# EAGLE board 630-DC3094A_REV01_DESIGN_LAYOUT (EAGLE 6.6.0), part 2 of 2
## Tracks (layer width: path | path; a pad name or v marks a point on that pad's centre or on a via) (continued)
N$30  (via drill 0.2) (continued)
  Bottom 0.15: v204.8,77 204.8,76.3 205,76.1 205.68,76.1
PFET_GATE
  Bottom 0.1: 21.3,73.4 M3.1 21.2,73.45 21.2,74.2 21.4,74.4 22.6,74.4 | 25.3,73.48 M2.1 | M1.1 29.3,73.52 29.3,74.2 29.1,74.4 25.5,74.4 25.3,74.2 | 25.3,74.2 M2.1 | M2.1 25.29,74.11 25.3,74.2 | 25.3,74.2 25.1,74.4 22.6,74.4 | 22.6,74.4 22.6,69.9 22.56,69.94 R10.1
  Bottom 0.15: R9.2 R10.1
PWRGD  (via drill 0.2)
  Top 0.1: U1.R1 129.3,54.8 129.3,57 128.9,57.4 v128.9,60.2 | v140.1,55.2 U1.A1 | U1.H1 v134.5,55.2
  Route2 0.1: v128.9,60.2 v133.7,60.2 v140.1,60.2 v160.4,60.2
  Route15 0.1: v140.1,60.2 v140.1,55.2 | v134.5,55.2 134.5,56.2 134.1,56.6 134.1,59.8 v133.7,60.2 | v160.4,60.2 160.41,77.2 161,77.8 161,81.05 TP8.TP
  Bottom 0.1: M4.1 165.4,77.05 R54.1 165.41,77.2 165.41,80.2 164.41,81.2 161.61,81.2 TP8.TP
  pour Route15 (no thermals): 161,78.6 160.9,79.2 160.6,79.7 161.4,79.7 161.1,79.2
  pour Bottom (no thermals): 163.81,81.2 163.21,81.3 162.81,81.6 162.81,80.8 163.21,81.1
PWRGD_A
  Top 0.152: J1.49 17.14,11.43 17.14,17.78 J7.49
PWRGD_B
  Top 0.152: J2.49 105.41,11.43 105.41,17.78 J8.49
PWRGD_C
  Top 0.152: J3.49 193.68,11.43 193.68,17.78 J9.49
REFM_A  (via drill 0.2)
  Top 0.1: U1.G1 v135.3,55.2 | 139,68.2 C10.2
  Top 0.15: v139,69 139,68.2
  Route15 0.1: v135.3,55.2 135.3,64.4 136.4,65.5 136.4,66.4 v139,69
REFM_B  (via drill 0.2)
  Top 0.1: U1.P1 v129.7,55.2
  Top 0.15: v129.9,69.1 C6.2
  Route15 0.1: v129.7,55.2 129.7,57 129.3,57.4 129.3,64.9 128.9,65.3 128.9,68.7 129.3,69.1 v129.9,69.1
REFM_C  (via drill 0.2)
  Top 0.1: U1.Z1 124.1,55.6 123.7,56 v123.3,56 | 115.8,68.08 C2.2
  Top 0.15: v115.9,69.2 C2.2
  Route2 0.1: v123.3,69.2 v115.9,69.2
  Route15 0.1: v123.3,56 v123.3,69.2
REFP_A  (via drill 0.2, 0.2 pad 0.25)
  Top 0.1: 138.9,66.32 C10.1
  Top 0.15: v138.9,65.5 138.9,66.32
  Route15 0.1: v135.7,57.2 135.7,62.3 v138.9,65.5
  Bottom 0.1: U1.G2 135.7,54 v135.7,57.2
  other vias: 135.3,53.6
REFP_B  (via drill 0.2, 0.2 pad 0.25)
  Top 0.1: U1.P2 130.1,54 130.1,56.9 129.7,57.3 129.7,58.8 v130.1,59.2 | 130.1,66.2 C6.1
  Top 0.15: v130.1,65.4 130.1,66.2
  Route15 0.1: v130.1,59.2 v130.1,65.4
  other vias: 129.7,53.6
REFP_C  (via drill 0.2)
  Top 0.1: U1.Z2 123.3,54.4 v123.3,55.2
  Top 0.15: v115.9,65.5 C2.1
  Route2 0.1: v123.3,55.2 122,55.2 121.8,55.4 v115.9,55.4
  Route15 0.1: v115.9,55.4 v115.9,65.5
RESETB  (via drill 0.2, 0.2 pad 0.25)
  Top 0.1: 233.65,75.4 233.68,75.37 SW1.SW1
  Top 0.15: TP7.TP 233.68,80.82 233.7,80.8 233.7,75.6 SW1.SW1 | v232.2,75.4 233.65,75.4 | R40.1 v144.5,65.5
  Route2 0.1: v128.1,56.4 v133.7,56.4 v139.3,56.4 v144.5,56.4 | J4.P$11 | v35.6,78.2 95.2,78.2 97.2,80.2 101,80.2 103,78.2 128.8,78.2 129.4,77.6 135,77.6 135.6,78.2 v144.5,78.2 230.6,78.2 TP7.TP
  Route2 0.15: J5.P$11 256.25,57.15 255.6,57.8 v232.2,57.8 | J4.P$11 11,57.8 v35.6,57.8
  Route15 0.1: U1.B2 139.3,54.1 139.7,54.5 139.7,56 v139.3,56.4 | v128.1,56.4 128.1,55.9 128.5,55.5 128.5,54 U1.T2 | U1.J2 134.1,54 134.1,56 v133.7,56.4 | v144.5,56.4 v144.5,65.5 v144.5,78.2 | v232.2,57.8 v232.2,75.4 | v35.6,57.8 v35.6,78.2
  Bottom 0.1: C15.2 232.2,73.23 v232.2,75.4
  other vias: 133.7,53.6 128.1,53.6 139.3,53.6
  pour Top (no thermals): 233.7,78.5 233.5,79.1 233.2,79.5 234.2,79.5 233.9,79.1
  pour Route2 (no thermals): 231.8,79.4 232.15,79.85 232.35,80.3 232.7,79.95 232.25,79.75
RUN_CH0  (via drill 0.2, 0.2 pad 0.23)
  Top 0.152: J1.11 65.41,11.43 65.41,17.78 J7.11
  Route2 0.1: v123.3,48.8 121.2,48.8 120.8,48.4 108.6,48.4 108.2,48.8 v102.4,48.8 v65.2,48.8
  Route15 0.1: U1.R7 128.5,49.2 123.7,49.2 v123.3,48.8 | v102.4,48.8 v102.4,65.4 | v65.2,48.8 65.2,20.05 J7.11
  Bottom 0.1: v102.4,65.4 R11.1
  other vias: 128.9,49.6
RUN_CH1  (via drill 0.2, 0.2 pad 0.25)
  Top 0.1: U1.W7 126.1,49.2 126.1,48.6 125.9,48.4 125.6,48.4 125.3,48.1 125.3,47 125,46.7 124.7,46.7 124.5,46.5 v124.5,44.8
  Route2 0.1: v63.8,44.6 v111.4,44.6 123.8,44.6 124,44.8 v124.5,44.8
  Route15 0.1: v111.4,44.6 v111.4,65.5 | v63.8,44.6 63.8,20.4 63.03,19.6 63.03,17.61 J7.12
  Bottom 0.1: R12.1 v111.4,65.5
  Bottom 0.152: J1.12 62.87,8.89 62.87,15.24 J7.12
  other vias: 126.5,49.6
RUN_CH2  (via drill 0.2, 0.2 pad 0.25)
  Top 0.152: J1.9 67.94,11.43 67.94,17.78 J7.9
  Route2 0.1: v123.3,46.4 122.7,45.8 v109.6,45.8 v66.73,45.8
  Route15 0.1: v109.6,45.8 v109.6,65.5 | v66.73,45.8 66.73,19.11 J7.9
  Bottom 0.1: U1.U7 126.9,49.2 126.9,48.6 126.7,48.4 126.3,48.4 126.1,48.2 126.1,47 125.9,46.8 125.3,46.8 124.9,46.4 v123.3,46.4 | v109.6,65.5 R13.1
  other vias: 127.3,49.6
RUN_CH3  (via drill 0.2, 0.2 pad 0.25)
  Route2 0.1: v123.3,45.6 122.9,45.2 v106,45.2 v67.4,45.2
  Route15 0.1: v106,45.2 v106,65.5 | v67.4,45.2 67.4,20.4 67.73,20 67.73,17.57 J7.10
  Bottom 0.1: U1.T7 127.7,49.2 127.7,47.8 125.9,46 124.9,46 124.5,45.6 v123.3,45.6 | v106,65.5 R14.1
  Bottom 0.152: J1.10 65.41,8.89 65.41,15.24 J7.10
  other vias: 128.1,49.6
RUN_CH4  (via drill 0.2, 0.2 pad 0.25)
  Top 0.152: J1.7 70.48,11.43 70.48,17.78 J7.7
  Route2 0.1: v69.2,50 v113.2,50 v120.9,50
  Route15 0.1: v113.2,50 v113.2,65.5 | v69.2,50 69.2,19.07 J7.7
  Bottom 0.1: R15.1 v113.2,65.5 | U1.W6 126.2,50.4 126.1,50.3 126.1,50.1 126,50 v120.9,50
  other vias: 126.5,50.4
RUN_CH5  (via drill 0.2, 0.2 pad 0.25)
  Route2 0.1: v122.5,48 v107.8,48 v69.8,48
  Route15 0.1: v107.8,48 v107.8,65.5 | v69.8,48 69.8,20.4 70.3,19.9 70.3,17.53 J7.8
  Bottom 0.1: U1.U6 126.9,50 126.3,50 126.1,49.8 126.1,49.4 125.9,49.2 125.5,49.2 125.3,49 125.3,48.6 125.1,48.4 124.5,48.4 124.1,48 v122.5,48 | v107.8,65.5 R16.1
  Bottom 0.152: J1.8 67.94,8.89 67.94,15.24 J7.8
  other vias: 127.3,50.4
RUN_CH6  (via drill 0.2, 0.2 pad 0.25)
  Top 0.152: J1.5 73.03,11.43 73.03,17.78 J7.5
  Route2 0.1: v120.1,52.4 v104.2,52.4 v71.33,52.4
  Route15 0.1: U1.T6 127.7,50.8 122.2,50.8 120.6,52.4 v120.1,52.4 | v104.2,52.4 v104.2,65.4 | v71.33,52.4 71.33,20.5 71.73,20.1 71.73,19.2 71.75,19.18 J7.5
  Bottom 0.1: v104.2,65.4 R17.1
  other vias: 128.1,50.4
RUN_CH7  (via drill 0.2, 0.2 pad 0.23)
  Route2 0.1: v121.7,50.4 v100.6,50.4 v71.9,50.4
  Route15 0.1: U1.R6 128.5,50 122.1,50 v121.7,50.4 | v100.6,50.4 v100.6,65.4 | v71.9,50.4 71.9,20.7 72.8,19.8 72.8,17.53 J7.6
  Bottom 0.1: v100.6,65.4 R18.1
  Bottom 0.152: J1.6 70.48,8.89 70.48,15.24 J7.6
  other vias: 128.9,50.4
RUN_CH8  (via drill 0.2, 0.2 pad 0.25)
  Top 0.152: J2.11 153.67,11.43 153.67,17.78 J8.11
  Route2 0.1: v140.4,23 140.4,21.6 v152.4,21.6 | U1.H7 137.3,46.8 137.9,46.8 138.2,46.5 138.2,45.9 v140.1,44
  Route15 0.1: v152.4,21.6 J8.11 | v140.1,44 140.1,33.5 140.4,33.2 v140.4,23
  Bottom 0.1: R26.1 v140.4,23
  other vias: 134.5,49.6
RUN_CH9  (via drill 0.2, 0.2 pad 0.25)
  Route2 0.1: U1.L7 131.7,49.2 131.7,46.2 132.1,45.8 132.1,45.2 v132.5,44.8
  Route15 0.1: v132.5,44.8 v132.5,30.4 132.5,20.5 133.6,19.4 133.6,15.9 134.3,15.2 151.09,15.2 J8.12
  Bottom 0.1: R27.1 132.5,29.39 v132.5,30.4
  Bottom 0.152: J2.12 151.13,8.89 151.13,15.24 J8.12
  other vias: 132.1,49.6
RUN_CH10  (via drill 0.2, 0.2 pad 0.25)
  Top 0.152: J2.9 156.21,11.43 156.21,17.78 J8.9
  Route2 0.1: v139.2,18 153.89,18 J8.9
  Route15 0.1: U1.K7 133.3,49.2 133.3,45.9 134.6,44.6 134.6,33.4 v137.6,30.4 137.6,20.8 138.7,19.7 138.7,18.5 v139.2,18
  Bottom 0.1: R28.1 137.6,29.5 v137.6,30.4
  other vias: 132.9,49.6
RUN_CH11  (via drill 0.2, 0.2 pad 0.25)
  Route2 0.1: v138.6,23 138.6,21.2 v153.8,21.2
  Route15 0.1: v153.8,21.2 153.8,17.65 J8.10 | v135.3,44 135.3,34.3 138.6,31 v138.6,23
  Bottom 0.1: R29.1 v138.6,23 | U1.J7 134.1,49.2 134.1,45.4 135.3,44.4 v135.3,44
  Bottom 0.152: J2.10 153.67,8.89 153.67,15.24 J8.10
  other vias: 133.7,49.6
RUN_CH12  (via drill 0.2, 0.2 pad 0.25)
  Top 0.152: J2.7 158.75,11.43 158.75,17.78 J8.7
  Route2 0.1: v134.1,20.4 156.13,20.4 J8.7
  Route15 0.1: v134.1,20.4 v134.1,30.4 132.9,31.6 132.9,45.2 v132.5,45.6
  Bottom 0.1: U1.L6 131.7,50 131.7,46.2 131.9,46 132.1,46 v132.5,45.6 | v134.1,30.4 134.1,29.49 R30.1
  other vias: 132.1,50.4
RUN_CH13  (via drill 0.2, 0.2 pad 0.25)
  Route2 0.1: v132.9,46.4 133,46.1 133.2,45.9 133.2,44.7 133.8,44.1 133.8,32.6 v136,30.4 137.6,28.8 v156.6,28.8
  Route15 0.1: v156.6,28.8 156.6,17.39 J8.8
  Bottom 0.1: U1.K6 132.5,50 132.5,46.8 v132.9,46.4 | R31.1 v136,30.4
  Bottom 0.152: J2.8 156.21,8.89 156.21,15.24 J8.8
  other vias: 132.9,50.4
RUN_CH14  (via drill 0.2, 0.2 pad 0.25)
  Top 0.152: J2.5 161.29,11.43 161.29,17.78 J8.5
  Route2 0.1: J8.5 159.95,19.05 158.2,20.8 136.8,20.8 v136.8,23
  Route15 0.1: v133.7,44.8 134.2,44.3 134.2,32.4 135.6,31 135.6,24.2 v136.8,23
  Bottom 0.1: U1.J6 133.3,50 133.3,45.2 v133.7,44.8 | v136.8,23 R32.1
  other vias: 133.7,50.4
RUN_CH15  (via drill 0.2, 0.2 pad 0.25)
  Route2 0.1: v142.2,23 142.2,22 159,22 161.2,19.8 161.2,17.69 J8.6
  Route15 0.1: v136.9,44 136.9,43.3 137.7,42.5 137.7,38.5 137.6,38.4 137.6,38 137.7,37.9 137.7,32.7 139,31.4 139,23.4 140,22.4 141.6,22.4 v142.2,23
  Bottom 0.1: R33.1 v142.2,23 | U1.H6 134.9,50 134.9,46.1 135.6,45.4 136,45.4 136.9,44.5 v136.9,44
  Bottom 0.152: J2.6 158.75,8.89 158.75,15.24 J8.6
  other vias: 134.5,50.4
RUN_CH16  (via drill 0.2)
  Top 0.1: U1.A7 v140.9,49.6
  Top 0.152: J3.11 241.94,11.43 241.94,17.78 J9.11
  Route2 0.1: v140.9,49.6 v155.9,49.6 194.37,49.6 194.56,49.4 205,49.4 205.2,49.2 v240.7,49.2
  Route15 0.1: v155.9,49.6 v155.9,65.5 | v240.7,49.2 240.7,19.15 J9.11
  Bottom 0.1: R42.1 155.96,66.46 155.9,66.4
  Bottom 0.15: 155.9,66.4 v155.9,65.5
RUN_CH17  (via drill 0.2)
  Top 0.1: U1.D7 138.1,49.2 149.4,49.2 150.2,50 v150.8,50
  Route2 0.1: v150.8,44.8 v239.8,44.8
  Route15 0.1: v150.8,65.5 v150.8,50 v150.8,44.8 | v239.8,44.8 239.8,17.41 J9.12
  Bottom 0.15: v150.8,65.5 R43.1
  Bottom 0.152: J3.12 239.4,8.89 239.4,15.24 J9.12
RUN_CH18  (via drill 0.2, 0.2 pad 0.25)
  Top 0.152: J3.9 244.47,11.43 244.47,17.78 J9.9
  Route2 0.1: U1.C7 138.9,49.2 v152.4,49.2 | v152.4,45.4 v243.2,45.4
  Route15 0.1: v152.4,65.5 v152.4,49.2 v152.4,45.4 | v243.2,45.4 243.2,19.09 J9.9
  Bottom 0.15: v152.4,65.5 R44.1
  other vias: 138.5,49.6
RUN_CH19  (via drill 0.2, 0.2 pad 0.25)
  Route2 0.1: v142.2,48.8 v154.2,48.8 | v154.2,46 v242.2,46
  Route15 0.1: v154.2,65.5 v154.2,48.8 v154.2,46 | U1.B7 139.7,50 141.7,50 142.2,49.5 v142.2,48.8 | v242.2,46 242.2,17.55 J9.10
  Bottom 0.1: 154.2,66.1 154.2,66.51 R45.1
  Bottom 0.15: v154.2,65.5 154.2,66.1
  Bottom 0.152: J3.10 241.94,8.89 241.94,15.24 J9.10
  other vias: 139.3,49.6
RUN_CH20  (via drill 0.2)
  Top 0.1: U1.D6 138.1,50.8 142.6,50.8 v143,51.2
  Top 0.152: J3.7 247.01,11.43 247.01,17.78 J9.7
  Route2 0.1: v144.6,35.4 v245.7,35.4
  Route15 0.1: v143.6,65.5 143.6,65 143,64.4 v143,51.2 143,47.4 144.6,45.8 144.6,42.7 144.5,42.6 144.5,42.2 144.6,42.1 v144.6,35.4 | v245.7,35.4 245.7,19.07 J9.7
  Bottom 0.15: v143.6,65.5 R46.1
RUN_CH21  (via drill 0.2, 0.2 pad 0.25)
  Route2 0.1: U1.C6 138.9,50 v145.4,50 149.6,50 150.1,50.5 151.7,50.5 152.2,50 194.97,50 195.16,49.8 205.2,49.8 205.4,49.6 v244.6,49.6
  Route15 0.1: v145.4,50 v145.4,65.5 | v244.6,49.6 244.6,17.69 J9.8
  Bottom 0.15: v145.4,65.5 R47.1
  Bottom 0.152: J3.8 244.47,8.89 244.47,15.24 J9.8
  other vias: 138.5,50.4
RUN_CH22  (via drill 0.2, 0.2 pad 0.25)
  Top 0.152: J3.5 249.56,11.43 249.56,17.78 J9.5
  Route2 0.1: U1.B6 139.7,50.8 v147.2,50.8 | v147.2,34.8 v248.2,34.8
  Route15 0.1: v147.2,65.5 v147.2,50.8 v147.2,34.8 | v248.2,34.8 248.2,19.17 J9.5
  Bottom 0.15: v147.2,65.5 R48.1
  other vias: 139.3,50.4
RUN_CH23  (via drill 0.2)
  Top 0.1: U1.A6 v140.9,50.4
  Route2 0.1: v140.9,50.4 v149,50.4 149.4,50.8 152.1,50.8 152.5,50.4 195.16,50.4 195.37,50.2 205.3,50.2 205.5,50 v247.16,50
  Route15 0.1: v149,50.4 v149,65.5 | v247.16,50 247.16,17.63 J9.6
  Bottom 0.15: v149,65.5 R49.1
  Bottom 0.152: J3.6 247.01,8.89 247.01,15.24 J9.6
SCL  (via drill 0.2, 0.2 pad 0.23, 0.2 pad 0.25)
  Route2 0.1: v125.1,81 102,81 101.6,81.4 96.6,81.4 96.2,81 62.2,81 62,81.2 58.7,81.2 TP1.TP | v125.3,56 v130.9,56 v136.9,56 147,56 147.4,55.6 v255.6,55.6 | J5.P$5 257.47,49.53 257.4,49.5
  Route2 0.15: v4.7,50.8 8.89,50.8 J4.P$5 | 257.4,49.5 v255.6,49.5
  Route15 0.1: U1.X2 125.3,54 v125.3,56 | v125.3,56 125.3,59.4 125.1,59.6 v125.1,81 | U1.E2 136.9,54.1 137.3,54.5 137.3,55.6 v136.9,56 | U1.M2 131.3,54.1 130.9,54.5 v130.9,56 | v125.3,56 125.3,56.2 | v255.6,49.5 v255.6,55.6 | 56.6,83.2 TP1.TP
  Route15 0.15: v4.7,50.8 4.7,77 11,83.3 17.6,83.3 18.59,82.31 J6.4 18.68,82.28 20.6,84.2 55.6,84.2 56.6,83.2 | 58.4,81.4 TP1.TP
  Bottom 0.1: R4.2 TP1.TP
  other vias: 136.9,53.6 125.7,53.6 131.3,53.6
  pour Route15 (no thermals): 56.6,83.2 57.05,82.85 57.6,82.7 57,82.2 56.9,82.7
  pour Route2 (no thermals): 61.1,81.2 60.4,81.3 60,81.5 60,80.9 60.4,81.1
  pour Bottom (no thermals): 58.4,78.6 58.6,79.1 58.9,79.5 57.95,79.5 58.25,79.1
SDA  (via drill 0.2)
  Top 0.1: U1.X1 v125.7,55.2 | v131.3,55.2 U1.M1 | U1.E1 v136.9,55.2
  Route2 0.1: v125.7,80.4 101.8,80.4 101.4,80.8 96.8,80.8 96.4,80.4 61,80.4 59.6,79 53.1,79 TP2.TP | v125.7,55.2 126.1,55.6 130.9,55.6 v131.3,55.2 131.7,55.6 136.5,55.6 v136.9,55.2 137.3,55.6 146.8,55.6 147.2,55.2 v254.9,55.2 | J5.P$7 257.7,52
  Route2 0.15: v5.4,53.3 8.1,53.3 8.6,52.8 9.4,52.8 9.43,52.77 J4.P$7 | 257.7,52 v254.9,52
  Route15 0.1: v125.7,55.2 v125.7,80.4 | v254.9,52 v254.9,55.2 | 47.2,81.3 TP2.TP
  Route15 0.15: v5.4,53.3 5.4,76.7 10.98,82.28 J6.2 16.62,82.28 17.6,81.3 27.8,81.3 30.1,83.6 44.9,83.6 47.2,81.3
  Bottom 0.1: R5.2 TP2.TP
  pour Route15 (no thermals): 47.8,81.3 48.6,81.4 49.2,81.7 49.2,80.9 48.6,81.2
  pour Bottom (no thermals): 50.8,78.6 50.6,79.1 50.3,79.5 51.3,79.5 51,79.1
  pour Route2 (no thermals): 52.7,79.4 52.15,79.8 51.65,79.95 52.15,80.45 52.3,79.95
SHARE_CLK  (via drill 0.2)
  Top 0.1: U1.B1 v139.3,55.2 | v133.7,55.2 U1.J1 | U1.T1 v128.1,55.2
  Top 0.15: R39.1 v146.3,65.5
  Route2 0.1: v128.1,55.2 128.5,54.8 133.3,54.8 v133.7,55.2 134.1,54.8 138.9,54.8 v139.3,55.2 139.7,54.8 140.3,54.8 140.7,55.2 v146.3,55.2 | J4.P$14 7.62,59.82 | v35,64.6 128,64.6 128.9,63.7 v146.3,63.7
  Route2 0.15: v146.3,72.4 171.2,72.4 172.3,71.3 v198.1,71.3 | v198.1,63.9 v227.1,63.9 | v227,60.5 255.1,60.5 255.6,61 259,61 J5.P$14 | 7.62,59.82 8.8,61 v35,61
  Route15 0.1: v146.3,55.2 v146.3,63.7 v146.3,65.5 v146.3,72.4 | TP6.TP 198.12,81.32 198.1,80.62 | v35,61 v35,64.6
  Route15 0.15: 198.1,80.62 v198.1,71.3 v198.1,63.9 | v227.1,63.9 v227,60.5
  pour Route15 (no thermals): 198.1,78.6 198.2,79.2 198.5,79.7 197.7,79.7 198,79.2
SPARE1
  Bottom 0.152: J1.48 17.14,8.89 17.14,15.24 J7.48
SPARE2
  Bottom 0.152: J1.50 14.61,8.89 14.61,15.24 J7.50
SPARE3
  Bottom 0.152: J1.52 12.06,8.89 12.06,15.24 J7.52
SPARE4  (via drill 0.2)
  Top 0.152: J1.47 19.68,11.43 19.68,17.78 J7.47
  Route2 0.1: J4.P$19 10.06,67.24 10,67.2 | v2.2,66.2 2.2,76.6 10.4,84.8 125,84.8 130.6,79.2 133.6,79.2 139.2,84.8 v257,84.8 | J7.47 18.39,19.05 17.2,20.2 17.2,27 4,40.2 v2.2,40.2
  Route2 0.15: 10,67.2 8.8,66.2 v2.2,66.2
  Route15 0.1: v257,84.8 257,68.12 J5.P$19 | v2.2,40.2 v2.2,66.2
SPARE5
  Top 0.152: J1.51 14.61,11.43 14.61,17.78 J7.51
SPARE6
  Bottom 0.152: J8.48 105.41,15.24 105.41,8.89 J2.48
SPARE7
  Bottom 0.152: J8.50 102.87,15.24 102.87,8.89 J2.50
SPARE8
  Bottom 0.152: J8.52 100.33,15.24 100.33,8.89 J2.52
SPARE9
  Top 0.152: J8.47 107.95,17.78 107.95,11.43 J2.47
SPARE10
  Top 0.152: J8.51 102.87,17.78 102.87,11.43 J2.51
SPARE11
  Bottom 0.152: J9.48 193.68,15.24 193.68,8.89 J3.48
SPARE12
  Bottom 0.152: J9.50 191.13,15.24 191.13,8.89 J3.50
SPARE13
  Bottom 0.152: J9.52 188.59,15.24 188.59,8.89 J3.52
SPARE14
  Top 0.152: J9.47 196.22,17.78 196.22,11.43 J3.47
SPARE15
  Top 0.152: J9.51 191.13,17.78 191.13,11.43 J3.51
USB_3.3V  (via drill 0.2)
  Top 0.1: C64.1 14.44,44.74 14.5,44.8
  Top 0.15: C64.1 J4.P$1 | 14.5,44.8 v14.5,45.5
  Route2 0.15: v29.7,75.4 31.2,76.8 31.2,79.6 35,83.4 124.6,83.4 129.8,78.2 134.2,78.2 139.6,83.6 253.2,83.6 v261.8,75
  Route15 0.15: v14.5,45.5 14.5,46.19 18.5,50.2 18.5,74.3 v19.6,75.4 | J5.P$1 258.85,44.45 259.2,44.8 259.2,45 259.8,45.6 260.9,45.6 261.8,46.5 v261.8,75
  Bottom 0.1: 20.59,75.39 M3.3 20.5,75.4
  Bottom 0.15: M3.3 M2.3 M1.3 28.73,75.4 v29.7,75.4 | J6.5 20.59,75.39 | v19.6,75.4 20.5,75.4
USB_5V
  Bottom 0.152: 16.59,72.98 16.59,74.63 R105.2
  Bottom 0.203: J6.1 16.59,72.98 14.22,70.61 C65.1 10.35,70.76 U4.4 | R105.2 R106.2
VDD25_A  (via drill 0.2)
  Top 0.1: U1.B3 U1.A3 v140.9,52.8
  Top 0.15: v140.9,69.1 C11.1
  Route15 0.1: v140.9,52.8 141.4,53.3 141.4,64.8 140.9,65.3 v140.9,69.1
VDD25_B  (via drill 0.2, 0.2 pad 0.25)
  Top 0.1: U1.H3 U1.J3 | 135.4,66.41 C7.1
  Top 0.15: v135.4,65.5 135.4,66.41
  Route15 0.1: U1.H3 134.9,53.2 134.9,56.2 135,56.3 135,57.1 134.9,57.2 134.9,65 v135.4,65.5
  other vias: 134.5,52.8
VDD25_C  (via drill 0.2)
  Top 0.1: U1.R3 U1.T3
  Top 0.15: v117.6,63.8 C3.1
  Route2 0.1: v127.7,63.8 v117.6,63.8
  Route15 0.1: U1.T3 127.7,53.2 v127.7,63.8
  other vias: 128.1,52.8
VDD33_A  (via drill 0.2, 0.2 pad 0.23)
  Top 0.1: U1.R4 U1.T4 | R6.2 R7.2 | 112.3,68.4 112,68.12 R6.2 | C4.1 R6.2
  Top 0.15: v111.9,69.2 112.3,68.8 112.3,68.4
  Route2 0.1: v126.9,69.7 115.5,69.7 v115,69.2 | 50.85,63.5 JP1.1 | 55.83,63.5 JP2.1
  Route2 0.15: 50.85,63.5 55.83,63.5 | v99.6,68.1 v54.6,68.1 v28.2,68.1
  Route15 0.1: v28.2,72.4 v28.2,68.1 | U1.T4 126.9,53.2 v126.9,69.7 | v102.4,69.2 102.4,76.3 v102.1,76.6 | 55.9,63.47 JP2.1
  Route15 0.15: v54.6,75.3 v54.6,68.1 54.6,67 55.9,65.7 55.9,63.47
  Bottom 0.1: v28.2,72.4 28.2,73.4 28.12,73.48 M1.2 | v99.61,68.11 v99.6,68.1 | R12.2 111.51,68.11 111.51,68.79 111.5,68.8 v111.9,69.2 | v115,69.2 R8.2 114.8,68.02 | v102.1,76.6 R56.2 | R5.1 | R4.1
  Bottom 0.15: R11.2 R18.2 v99.61,68.11 | R11.2 R17.2 R14.2 R16.2 R13.2 R12.2 R15.2 R8.2 | R11.2 v102.4,69.2 | R5.1 v54.6,75.3 R4.1
  other vias: 128.1,52
VDD33_B  (via drill 0.2, 0.2 pad 0.25)
  Top 0.1: U1.H4 U1.J4
  Top 0.15: R25.2 v133.7,69.1 137.3,69.1 C8.1 | R24.2 v128,69.1
  Top 0.2: R23.2 R25.2
  Route2 0.1: 63.55,63.5 JP3.1 | 68.53,63.5 JP4.1
  Route2 0.15: v24,67.2 v63.5,67.2 123.4,67.2 125.3,69.1 v128,69.1 128.5,69.6 133.2,69.6 v133.7,69.1 134.2,69.6 v151.8,69.6 | 63.55,63.5 68.53,63.5 | v142.2,26.8 v151.8,26.8
  Route15 0.1: U1.J4 133.3,52.4 133.3,60.2 v132.9,60.6 | 68.6,63.47 JP4.1
  Route15 0.15: v24,72.2 v24,67.2 | v132.9,60.6 133.3,61 133.3,68.7 v133.7,69.1 | v151.8,26.8 v151.8,69.6 | v63.5,67.2 JP3.1
  Bottom 0.1: M2.2 23.99,72.21 v24,72.2 | R22.2 132.2,59.9 v132.9,60.6 | R32.2 | 137.81,25.71 137.8,25.7 R33.2 | R30.2 137.71,27.69 137.8,27.6
  Bottom 0.15: R27.2 R30.2 R31.2 R28.2 137.8,27.6 137.8,25.7 R32.2 | R33.2 R26.2 R29.2 137.81,25.71 | R33.2 v142.2,26.8
  other vias: 133.7,52
VDD33_C  (via drill 0.2)
  Top 0.1: 220.96,75.4 LED5.P | U1.B4 U1.A4 v140.9,52 | 205.6,75.4 205.72,75.4 LED3.P 205.62,75.42 205.6,75.4 | 213.2,75.4 213.34,75.4 LED4.P 213.22,75.42 213.2,75.4
  Top 0.15: 205.6,75.4 v204.8,75.4 | 213.34,75.4 v214.3,75.4 | v221.9,75.4 220.96,75.4 | R38.2 R37.2 R39.2 R40.2 | R40.2 C12.1 | R40.2 R47.2 v145.4,69.1 | LED2.P 160.9,75.42 160.9,75.4 v157.2,75.4
  Route2 0.1: 81.23,63.5 JP6.1 | 76.25,63.5 JP5.1
  Route2 0.15: v20.1,66.4 v81.2,66.4 | 76.25,63.5 81.23,63.5 | v221.9,75.4 v214.3,75.4 v204.8,75.4 v164.3,75.4 v157.2,75.4 103.2,75.4 103,75.2 v81.2,75.2
  Route15 0.1: v140.9,52 141.8,52.9 141.8,64.8 141.3,65.3 141.3,68.6 v141.8,69.1 | 81.2,63.53 JP6.1
  Route15 0.15: v20.1,72.2 v20.1,66.4 | v157.2,68.1 v157.2,75.4 | v81.2,75.2 v81.2,66.4 81.2,63.53 | v222.8,62.9 222.8,74.6 v221.9,75.4
  Bottom 0.1: v20.1,72.2 20.1,73.1 19.92,73.28 M3.2 | U2.5 214.3,73.09 | U3.5 221.9,73.11 | R42.2 156,68.11 | R121.2 R120.2 R119.2 R118.2 R117.2 221.8,62.9 v222.8,62.9
  Bottom 0.15: v164.3,75.4 R54.2 | 214.3,73.09 v214.3,75.4 | 221.9,73.11 v221.9,75.4 | R42.2 R45.2 R44.2 R43.2 R49.2 R48.2 R47.2 v145.4,69.1 R47.2 R46.2 R41.2 v141.8,69.1 | 156,68.11 156.19,68.11 156.2,68.1 v157.2,68.1 | C66.1 216.92,72.88 216.8,73 214.39,73 U2.5
  Bottom 0.2: 145.4,68.22 R47.2
VIN  (via drill 0.2)
  Route2 0.1: v19.6,68.7 v3.4,68.7
  Route2 0.61: J3.26 221.19,5.9 182.1,5.9 179.5,8.5 173.5,8.5 170.9,5.9 136.31,5.9 J2.26 132.93,5.9 93.19,5.9 90.6,8.5 84.6,8.5 82,5.9 48.1,5.9 46.38,7.62 J1.26
  Route15 0.1: v3.4,68.7 3.4,43.6 3.8,43.2 3.8,35.6 TP9.TP
  Route15 0.15: J1.26 44.53,5.8 9.04,5.8 7.35,7.51 7.33,28.86 3.8,32.4 3.8,35.6
  Route15 0.203: 3.8,35.6 3.81,35.61 TP9.TP
  Route15 0.61: J3.26 221.09,5.8 181.9,5.8 179.4,8.3 173.6,8.3 171.1,5.8 136.41,5.8 J2.26 132.83,5.8 92.9,5.8 90.4,8.3 84.8,8.3 82.3,5.8 48.15,5.8 J1.26
  Bottom 0.1: v19.6,68.7 20.3,68.7 20.4,68.8 20.46,68.74 R9.1 | R1.1 J7.25 | R34.1 J9.25
  Bottom 0.305: J1.26 J1.25 J7.26 J7.25 | J9.25 J9.26 J3.25 J3.26 | J8.25 R19.1 J2.26 J2.25 J8.26 J8.25
  Bottom 0.61: J1.26 48.39,5.59 82.3,5.59 84.84,8.13 90.42,8.13 92.96,5.59 132.59,5.59 J2.26 136.65,5.59 171.2,5.59 173.74,8.13 179.58,8.13 182.12,5.59 220.85,5.59 J3.26
  pour Route15 (no thermals): 3.8,33 3.9,33.5 4.25,34 3.35,34 3.7,33.5
  pour Route15 (no thermals): 3.8,38.1 3.7,37.6 3.4,37.1 4.2,37.1 3.9,37.6
VIN_A  (via drill 0.2, 0.2 pad 0.25)
  Top 0.15: v119.4,49.2 C1.1
  Route2 0.1: v119.4,49.2 v47.4,49.2
  Route15 0.1: v47.4,49.2 v47.4,24.8
  Bottom 0.1: U1.R5 128.5,51.6 120.4,51.6 119.4,50.6 v119.4,49.2 | v47.4,24.8 46.48,24.8 R1.2
  other vias: 128.9,51.2
VIN_B  (via drill 0.2, 0.2 pad 0.25)
  Top 0.1: C5.1 134.9,59.4 135,59.4 | U1.H5 134.9,51.6 134.9,55.6 136.1,56.8 136.1,58.9 135.6,59.4 135,59.4 | 135,59.4 C5.1 | C5.1 134.5,59.7 v134.5,60.9
  Route2 0.1: v134.5,60.9 133.9,60.9 133.7,61.1 131.9,61.1 131.4,60.6 v119,60.6 | v119,24 133,24 v133.6,24.6
  Route15 0.1: v119,60.6 v119,24
  Bottom 0.1: v133.6,24.6 134.54,24.6 R19.2
  other vias: 134.5,51.2
VIN_C  (via drill 0.2)
  Top 0.1: U1.A5 v140.9,51.2 | 154.6,51.6 154.7,51.6 154.8,51.7 C9.1 154.7,51.7 154.6,51.6
  Top 0.15: 154.6,51.6 v153.6,51.6
  Route2 0.1: v140.9,51.2 141.3,51.2 141.9,51.8 142.3,51.8 142.5,52 152.8,52 153.2,51.6 v153.6,51.6 202.97,51.6 203.16,51.4 204.76,51.4 204.97,51.6 v222.9,51.6
  Route15 0.1: v222.9,51.6 v222.9,25.8
  Bottom 0.1: v222.9,25.8 222.9,24.77 R34.2
VIN_EN_A  (via drill 0.2, 0.2 pad 0.23)
  Top 0.1: R109.2 251.23,48.77 251.2,48.8 v250.2,48.8
  Top 0.152: J1.3 75.56,11.43 75.56,17.78 J7.3
  Route2 0.1: U1.W5 126.1,50.8 125.3,50.8 124.5,51.6 122.7,51.6 122.3,52 v115,52 v74.23,52 | v250.2,48.8 v164,48.8 | v164,61 136.6,61 136.2,61.4 131.4,61.4 131,61.8 v115,61.8
  Route15 0.1: v115,52 v115,61.8 v115,65.5 | v74.23,52 74.23,19.11 J7.3 | v164,48.8 v164,61
  Bottom 0.1: v115,65.5 R8.1
  other vias: 126.5,51.2
VIN_EN_B  (via drill 0.2, 0.2 pad 0.25)
  Top 0.1: 133.6,66.41 R25.1 | v249.2,47 R110.2
  Top 0.15: v132.8,65.4 133.4,65.4 133.6,65.6 133.6,66.41
  Top 0.152: J2.3 163.83,11.43 163.83,17.78 J8.3
  Route2 0.1: v132.8,65.4 133.8,66.4 v162.2,66.4 187.2,66.4 187.4,66.2 v247.6,66.2
  Route15 0.1: U1.L5 131.7,51.6 131.7,52.4 132.5,53.2 132.5,65.1 v132.8,65.4 | J8.3 162.56,20.64 162.2,21 v162.2,66.4 | v247.6,66.2 247.6,51.8 249.2,50.2 v249.2,47
  other vias: 132.1,51.2
VIN_EN_C  (via drill 0.2, 0.2 pad 0.25)
  Top 0.1: U1.D5 138.1,51.6 138.7,51.6 138.9,51.8 138.9,52.9 139.2,53.2 v142.2,53.2 | R111.2 251.42,43.92 v251.4,43.9
  Top 0.152: J3.3 252.09,11.43 252.09,17.78 J9.3 | v251.4,43.9 251.4,45.17 R111.2
  Route2 0.1: v251.4,53.2 v142.2,53.2
  Route2 0.152: J9.3 250.82,19.44 250.76,19.5 250.76,20.51 251.33,21.08 v251.4,43.9
  Route15 0.1: v142.2,53.2 142.2,65.1 v141.8,65.5 | v251.4,43.9 v251.4,53.2
  Bottom 0.15: v141.8,65.5 R41.1
  other vias: 137.7,51.2
VIN_SNS_A  (via drill 0.2, 0.2 pad 0.23)
  Top 0.1: U1.T5 127.7,50.8 125.5,50.8 125.3,50.6 125.3,48.6 125.1,48.4 124.7,48.4 124.5,48.2 124.5,47.8 124.3,47.6 122.1,47.6 v121.7,47.2
  Route2 0.1: v121.7,47.2 v74.8,47.2
  Route15 0.1: v74.8,47.2 74.8,20.4 75.4,19.8 75.4,17.55 J7.4 | v80.44,11.2 80.44,10.2 79.03,8.8 75.47,8.8 J1.4
  Bottom 0.1: R112.2 v80.44,11.2
  Bottom 0.152: J1.4 73.03,8.89 73.03,15.24 J7.4
  other vias: 128.1,51.2
VIN_SNS_B  (via drill 0.2, 0.2 pad 0.25)
  Route2 0.1: U1.J5 134.1,51.6 136.5,51.6 136.9,52 138.5,52 138.9,52.4 141.2,52.4 141.5,52.7 141.5,53.5 141.8,53.8 v161.4,53.8
  Route15 0.1: v161.4,53.8 161.4,17.67 J8.4 | v168.6,11 168.6,10 167.4,8.8 163.74,8.8 J2.4
  Bottom 0.1: R113.2 v168.6,11
  Bottom 0.152: J2.4 161.29,8.89 161.29,15.24 J8.4
  other vias: 133.7,51.2
VIN_SNS_C  (via drill 0.2, 0.2 pad 0.25)
  Route2 0.1: v142.2,52.4 203.37,52.4 203.56,52.2 204.26,52.2 204.76,52.7 v250.2,52.7
  Route15 0.1: U1.B5 139.7,51.6 141.4,51.6 v142.2,52.4 | v250.2,52.7 250.2,49.8 250.7,49.3 250.7,48.5 249.8,47.6 249.8,17.57 J9.4 | v256.8,11 256.8,10 255.6,8.8 252,8.8 J3.4
  Bottom 0.1: R114.2 256.8,12.6 v256.8,11
  Bottom 0.152: J3.4 249.56,8.89 249.56,15.24 J9.4
  other vias: 139.3,51.2
VIN_SNS_X  (via drill 0.2)
  Route2 0.1: v256.8,15.6 256.8,39.4 260.3,42.9 260.3,44.4 J5.P$2
  Route2 0.15: v262.4,75.4 253.6,84.2 139.4,84.2 133.9,78.7 130.2,78.7 124.7,84.2 v10.8,84.2 | v4,44.4 7.57,44.4 J4.P$2
  Route15 0.1: v81.83,14.2 v167.2,14.2 v255.76,14.2
  Route15 0.15: J5.P$2 261.85,44.45 262.4,45 v262.4,75.4 | v10.8,84.2 4,77.4 v4,44.4
  Bottom 0.1: 256.8,14.2 v256.8,15.6 | R112.1 v81.83,14.2 | v167.2,14.2 R113.1 | v255.76,14.2 256.8,14.2 | 256.8,14.2 R114.1
VSNSM0  (via drill 0.2)
  Top 0.1: U1.Z5 v123.3,51.2 | v21,30.4 21.04,29.33 C17.1 R58.2
  Route2 0.1: v120.9,52.8 v21,52.8
  Route15 0.1: v123.3,51.2 122.6,51.2 121,52.8 v120.9,52.8 | v21,52.8 v21,30.4
  Bottom 0.1: C17.1 21,29.6 v21,30.4
VSNSM1  (via drill 0.2)
  Top 0.1: v28.6,30.4 28.6,29.56 R60.2
  Route2 0.1: U1.X6 125.3,50 123,50 122.2,50.8 68.6,50.8 68.2,50.4 v28.6,50.4
  Route15 0.1: v28.6,50.4 v28.6,30.4
  Bottom 0.1: C19.1 28.6,29.6 v28.6,30.4
  other vias: 125.7,50.4
VSNSM2  (via drill 0.2)
  Top 0.1: v33.63,30.4 33.63,29.27 C21.1 R62.2
  Route2 0.1: U1.Y8 124.4,48.8 123.2,47.6 122.9,47.6 v122.5,47.2 | v121.8,38.7 40.7,38.7 40.6,38.6 39.8,38.6 39.7,38.7 v33.63,38.7
  Route15 0.1: v33.63,38.7 v33.63,30.4 | v122.5,47.2 121.8,46.5 v121.8,38.7
  Bottom 0.1: R62.2 33.66,29.58 33.63,29.6 v33.63,30.4 | 33.63,29.52 R62.2 | C21.1 R62.2
  other vias: 124.9,48.8
VSNSM3  (via drill 0.2)
  Top 0.1: C23.1 36.23,29.29 v36.23,30.4 36.23,29.54 R64.2
  Route2 0.1: U1.X8 125.3,48.4 124.6,48.4 122.8,46.6 v36.23,46.6
  Route15 0.1: v36.23,46.6 v36.23,30.4
  Bottom 0.1: R64.2 C23.1 36.2,29.56 36.23,29.6 v36.23,30.4
  other vias: 125.7,48.8
VSNSM4  (via drill 0.2)
  Top 0.1: v41.2,30.4 41.23,29.54 R66.2
  Route2 0.1: v124.6,40.4 v41.2,40.4
  Route15 0.1: v41.2,40.4 v41.2,30.4 | U1.Y10 124.9,42.4 124.6,42.1 v124.6,40.4
  Bottom 0.1: C25.1 41.34,29.6 41.2,29.6 v41.2,30.4
  other vias: 124.9,47.2
VSNSM5  (via drill 0.2)
  Top 0.1: v56.4,30.4 56.4,29.33 C27.1 R68.2
  Route2 0.1: U1.T9 126.5,46.4 126.5,43.6 125.9,43 v56.4,43
  Route15 0.1: v56.4,43 v56.4,30.4
  Bottom 0.1: C27.1 R68.2 | 56.44,29.58 R68.2 | R68.2 56.52,29.62 56.4,29.7 v56.4,30.4
  other vias: 128.1,48
VSNSM6  (via drill 0.2)
  Top 0.1: v59,30.4 59,29.52 R70.2
  Route2 0.1: v127.3,46.4 126.8,45.9 126.8,43.5 125.9,42.6 v59,42.6
  Route15 0.1: v59,42.6 v59,30.4 | U1.R10 128.1,47.2 v127.3,46.4
  Bottom 0.1: C29.1 59,29.6 v59,30.4
  other vias: 128.9,47.2
VSNSM7  (via drill 0.2)
  Top 0.1: v61.6,30.4 61.6,29.54 R72.2
  Route2 0.1: v126.4,42.2 v61.6,42.2
  Route15 0.1: U1.T8 127.7,48.4 127.7,47.8 126.5,46.6 126.5,42.8 126.4,42.7 v126.4,42.2 | v61.6,42.2 v61.6,30.4
  Bottom 0.1: C31.1 61.59,29.56 61.6,29.6 v61.6,30.4
  other vias: 128.1,48.8
VSNSM8  (via drill 0.2, 0.2 pad 0.25)
  Top 0.1: 109.52,29.2 R74.2
  Top 0.15: v110.4,29.2 109.52,29.2
  Route15 0.1: v110.4,46.2 v110.4,29.2
  Bottom 0.1: C33.1 109.35,29.25 109.6,29.2 v110.4,29.2 | U1.P5 129.3,50.8 124.5,50.8 124.2,50.5 122.7,50.5 122.4,50.8 121.3,50.8 121.1,50.6 120.6,50.6 120.2,50.2 120.2,48.2 118.2,46.2 v110.4,46.2
  other vias: 129.7,51.2
VSNSM9  (via drill 0.2)
  Top 0.1: U1.M6 130.9,50 130.9,46.8 v130.5,46.4 | 117.14,29.2 R76.2
  Top 0.15: v117.8,29.2 117.14,29.2
  Route2 0.1: v130.5,29.2 v117.8,29.2
  Route15 0.1: v130.5,46.4 v130.5,29.2
  Bottom 0.1: v117.8,29.2 116.89,29.2 C35.1
  other vias: 131.3,50.4
VSNSM10  (via drill 0.2)
  Top 0.1: 121.9,29.9 121.9,29.52 R78.2 121.92,29.88 121.9,29.9
  Top 0.15: 121.9,29.9 v121.9,30.6
  Route2 0.1: v130.1,30.6 v121.9,30.6
  Route15 0.1: U1.N8 130.1,48.4 v130.1,30.6
  Bottom 0.1: v121.9,30.6 121.9,29.27 C37.1
  other vias: 130.5,48.8
VSNSM11  (via drill 0.2)
  Top 0.1: 124.76,29.8 R80.2
  Top 0.15: v125.4,29.8 124.76,29.8
  Route2 0.1: v131.3,29.8 v125.4,29.8
  Route15 0.1: U1.M8 130.9,48.4 130.9,46.4 131.3,46 v131.3,29.8
  Bottom 0.1: v125.4,29.8 125.01,29.8 C39.1
  other vias: 131.3,48.8
VSNSM12  (via drill 0.2)
  Top 0.1: v131.3,28.6 130.44,28.6 R82.2
  Route15 0.1: v131.7,45.6 131.7,29 v131.3,28.6
  Bottom 0.1: U1.N10 131.3,46.4 131.3,46 v131.7,45.6 | C41.1 130.25,28.6 v131.3,28.6
  other vias: 130.5,47.2
VSNSM13  (via drill 0.2)
  Top 0.1: U1.J9 134.1,47.6 134.1,45.8 135,44.9 135.6,44.9 136.1,44.4 v136.1,44 | 144.6,29.68 R84.2
  Top 0.15: v144.6,30.6 144.6,29.68
  Route2 0.1: v137.1,35.4 v143.8,35.4
  Route15 0.1: v136.1,44 136.1,43.3 137.1,42.3 v137.1,35.4 | v143.8,35.4 143.8,31.4 v144.6,30.6
  Bottom 0.1: C43.1 144.6,29.6 v144.6,30.6
VSNSM14  (via drill 0.2)
  Top 0.1: U1.H10 v134.5,46.4 | 147.2,29.62 R86.2 147.42,29.4
  Top 0.15: v147.2,33.6 147.2,29.62
  Route2 0.1: v134.5,46.4 135.3,45.6 136.5,45.6 137.2,44.9 138.1,44.9 139.3,43.7 v139.3,43.2 | v139.5,33.6 v147.2,33.6
  Route15 0.1: v139.3,43.2 139.3,39.7 139.2,39.6 139.2,39.2 139.5,38.9 v139.5,33.6
  Bottom 0.1: C45.1 147.45,29.25 147.6,29.4 147.42,29.4 R86.2 147.32,29.58 147.2,29.7 v147.2,33.6
VSNSM15  (via drill 0.2)
  Top 0.1: C47.1 150.21,29.6 150.21,29.41 149.8,29.6 149.96,29.6 | 150,29.6 149.96,29.6 | 149.96,29.6 R88.2
  Top 0.15: v149.8,30.6 149.8,29.6
  Route2 0.1: U1.J8 134.1,48.4 134.1,46.1 134.4,45.8 134.6,45.8 135.2,45.2 136.2,45.2 136.5,44.9 136.5,34.6 138.3,32.8 v149.8,32.8
  Route15 0.1: v149.8,32.8 v149.8,30.6
  Bottom 0.1: R88.2 C47.1 150.05,29.25 149.8,29.5 v149.8,30.6
  other vias: 133.7,48.8
VSNSM16  (via drill 0.2)
  Top 0.1: 197.49,29.25 197.13,29.6 197.46,29.6 R90.2
  Top 0.15: 197.13,29.6 v195.8,29.6
  Route2 0.1: v143.8,51.2 152.4,51.2 152.8,50.8 v195.8,50.8
  Route15 0.1: v195.8,50.8 v195.8,29.6
  Bottom 0.1: U1.G5 135.7,51.6 143.4,51.6 v143.8,51.2 | C49.1 197.12,29.6 v195.8,29.6
  other vias: 135.3,51.2
VSNSM17  (via drill 0.2)
  Top 0.1: 205.01,29.6 R92.2
  Top 0.15: v203.4,29.6 205.01,29.6
  Route2 0.1: v142.2,51.2 142.6,51.6 152.6,51.6 153,51.2 v202.56,51.2
  Route15 0.1: U1.E6 137.3,50.8 141.8,50.8 v142.2,51.2 | v202.56,51.2 202.56,50.73 203.4,49.93 v203.4,29.6
  Bottom 0.1: C51.1 204.92,29.6 v203.4,29.6
  other vias: 136.9,50.4
VSNSM18  (via drill 0.2)
  Top 0.1: v210.16,30.6 210.16,29.52 R94.2
  Route2 0.1: U1.F8 137.3,47.6 138.1,47.6 138.9,46.8 v210.16,46.8
  Route15 0.1: v210.16,46.8 v210.16,30.6
  Bottom 0.1: 210.16,29.6 v210.16,30.6
  Bottom 0.15: C53.1 210.16,29.6
  other vias: 136.1,48.8
VSNSM19  (via drill 0.2)
  Top 0.1: v212.76,30.6 212.76,29.54 R96.2
  Route2 0.1: v142,37.6 v212.76,37.6
  Route15 0.1: U1.E8 137.3,48.4 137.9,48.4 138.1,48.2 138.1,47.7 139.1,46.7 139.1,46.3 139.7,45.7 140.8,45.7 142,44.5 v142,37.6 | v212.76,37.6 v212.76,30.6
  Bottom 0.1: 212.76,29.7 v212.76,30.6
  Bottom 0.15: C55.1 212.76,29.7
  other vias: 136.9,48.8
VSNSM20  (via drill 0.2)
  Top 0.1: U1.F10 v136.1,46.4 | v217.76,30.6 217.76,29.54 R98.2
  Route2 0.1: v139.7,39.4 v217.76,39.4
  Route15 0.1: v136.1,46.4 136.1,46 136.7,45.4 138,45.4 139.7,43.7 v139.7,39.4 | v217.76,39.4 v217.76,30.6
  Bottom 0.1: 217.76,29.6 v217.76,30.6
  Bottom 0.15: C57.1 217.76,29.6
VSNSM21  (via drill 0.2)
  Top 0.1: R100.2 232.94,29.35 232.82,29.35 232.76,29.4 v231.9,29.4
  Route2 0.1: v142.8,41.2 v231.9,41.2
  Route15 0.1: U1.B9 140.5,46.8 140.8,46.8 142.8,44.8 v142.8,41.2 | v231.9,41.2 v231.9,29.4
  Bottom 0.1: v231.9,29.4 232.89,29.4 C59.1
  other vias: 139.3,48
VSNSM22  (via drill 0.2)
  Top 0.1: R102.2 235.47,29.4 v234.56,29.4 | U1.A10 v140.1,46.4
  Route2 0.1: v140.1,46.4 v234.56,46.4
  Route15 0.1: v234.56,46.4 v234.56,29.4
  Bottom 0.1: v234.56,29.4 235.43,29.4 C61.1
VSNSM23  (via drill 0.2)
  Top 0.1: R104.2 238.07,29.5 237.97,29.4 v237.2,29.4 | U1.B8 139.7,48.4 140.6,48.4 141.2,47.8 143.2,47.8 v143.8,47.2
  Route2 0.1: v145,42.4 v237.2,42.4
  Route15 0.1: v143.8,47.2 145,46 v145,42.4 | v237.2,42.4 v237.2,29.4
  Bottom 0.1: v237.2,29.4 237.97,29.4 C63.1
  other vias: 139.3,48.8
VSNSM_CH0  (via drill 0.2)
  Top 0.1: R58.1 20.74,27.9 20.64,27.8 v19.8,27.8
  Route15 0.1: v19.8,27.8 19.8,17.63 J7.46
  Bottom 0.152: J1.46 19.68,8.89 19.68,15.24 J7.46
VSNSM_CH1  (via drill 0.2)
  Top 0.1: R60.1 28.34,27.9 28.23,27.8 v27.4,27.8
  Route15 0.1: v27.4,27.8 27.4,17.65 J7.40
  Bottom 0.152: J1.40 27.3,8.89 27.3,15.24 J7.40
VSNSM_CH2  (via drill 0.2)
  Top 0.1: R62.1 33.54,27.9 33.44,27.8 v32.6,27.8
  Route15 0.1: v32.6,27.8 32.6,17.53 J7.36
  Bottom 0.152: J1.36 32.38,8.89 32.38,15.24 J7.36
VSNSM_CH3  (via drill 0.2)
  Top 0.1: R64.1 36.14,27.9 36.03,27.8 v35.2,27.8
  Route15 0.1: v35.2,27.8 35.2,17.47 J7.34
  Bottom 0.152: J1.34 34.92,8.89 34.92,15.24 J7.34
VSNSM_CH4  (via drill 0.2)
  Top 0.1: v42.23,27.8 41.38,27.8 R66.1
  Route15 0.1: J7.30 41.34,16.51 42.23,17.4 v42.23,27.8
  Bottom 0.152: J1.30 40.01,8.89 40.01,15.24 J7.30
VSNSM_CH5  (via drill 0.2)
  Top 0.1: v55.44,27.8 56.41,27.8 R68.1
  Route15 0.1: J7.18 56.33,16.51 55.44,17.4 v55.44,27.8
  Bottom 0.152: J1.18 55.24,8.89 55.24,15.24 J7.18
VSNSM_CH6  (via drill 0.2)
  Top 0.1: v58,27.8 58.95,27.8 R70.1
  Route15 0.1: J7.16 58.92,16.51 58,17.4 v58,27.8
  Bottom 0.152: J1.16 57.78,8.89 57.78,15.24 J7.16
VSNSM_CH7  (via drill 0.2)
  Top 0.1: v60.63,27.8 61.49,27.8 R72.1
  Route15 0.1: J7.14 61.52,16.51 60.63,17.4 v60.63,27.8
  Bottom 0.152: J1.14 60.33,8.89 60.33,15.24 J7.14
VSNSM_CH8  (via drill 0.2)
  Top 0.1: R74.1 109.1,27.9 109,27.8
  Top 0.15: 109,27.8 v108,27.8
  Route15 0.1: v108,27.8 108,17.73 J8.46
  Bottom 0.152: J2.46 107.95,8.89 107.95,15.24 J8.46
VSNSM_CH9  (via drill 0.2)
  Top 0.1: 116.74,27.8 R76.1
  Top 0.15: v115.8,27.8 116.74,27.8
  Route15 0.1: J8.40 116.79,16.51 115.8,17.5 v115.8,27.8
  Bottom 0.152: J2.40 115.57,8.89 115.57,15.24 J8.40
VSNSM_CH10  (via drill 0.2)
  Top 0.1: R78.1 121.9,27.9 121.8,27.8
  Top 0.15: 121.8,27.8 v121,27.8
  Route15 0.1: v121,27.8 121,17.43 J8.36
  Bottom 0.152: J2.36 120.65,8.89 120.65,15.24 J8.36
VSNSM_CH11  (via drill 0.2)
  Top 0.1: R80.1 124.3,27.9 124.2,27.8
  Top 0.15: 124.2,27.8 v123.5,27.8
  Route15 0.1: v123.5,27.8 123.5,17.47 J8.34
  Bottom 0.152: J2.34 123.19,8.89 123.19,15.24 J8.34
VSNSM_CH12  (via drill 0.2)
  Top 0.1: R82.1 129.54,27.86 129.6,27.8
  Top 0.15: 129.6,27.8 v130.5,27.8
  Route15 0.1: v130.5,27.8 130.5,17.47 J8.30
  Bottom 0.152: J2.30 128.27,8.89 128.27,15.24 J8.30
VSNSM_CH13  (via drill 0.2)
  Top 0.1: R84.1 144.5,27.9 144.4,28 v143.7,28
  Route15 0.1: v143.7,28 143.7,25.4 143.8,25.3 143.8,24.6 143.7,24.5 143.7,17.59 J8.18
  Bottom 0.152: J2.18 143.51,8.89 143.51,15.24 J8.18
VSNSM_CH14  (via drill 0.2)
  Top 0.1: R86.1 147.1,27.9 147,28 v146.3,28
  Route15 0.1: v146.3,28 146.3,17.53 J8.16
  Bottom 0.152: J2.16 146.05,8.89 146.05,15.24 J8.16
VSNSM_CH15  (via drill 0.2)
  Top 0.1: v148.9,28 149.86,28 R88.1
  Route15 0.1: J8.14 148.9,17.47 v148.9,28
  Bottom 0.152: J2.14 148.59,8.89 148.59,15.24 J8.14
VSNSM_CH16  (via drill 0.2)
  Top 0.1: R90.1 197.49,27.72 197.47,27.7
  Top 0.15: 197.47,27.7 v197.47,26.6
  Route15 0.1: v197.47,26.6 197.47,20.9 196.37,19.8 196.37,17.63 J9.46
  Bottom 0.152: J3.46 196.22,8.89 196.22,15.24 J9.46
VSNSM_CH17  (via drill 0.2)
  Top 0.1: R92.1 205.1,27.64 205.06,27.6
  Top 0.15: 205.06,27.6 v205.06,26.6
  Route15 0.1: v205.06,26.6 205.06,20.9 203.97,19.8 203.97,17.65 J9.40
  Bottom 0.152: J3.40 203.84,8.89 203.84,15.24 J9.40
VSNSM_CH18  (via drill 0.2)
  Top 0.1: R94.1 210.19,27.62 210.16,27.6
  Top 0.15: 210.16,27.6 v210.16,26.6
  Route15 0.1: v210.16,26.6 210.16,20.8 209.16,19.8 209.16,17.53 J9.36
  Bottom 0.152: J3.36 208.91,8.89 208.91,15.24 J9.36
VSNSM_CH19  (via drill 0.2)
  Top 0.1: R96.1 212.72,27.64 212.76,27.6
  Top 0.15: 212.76,27.6 v212.76,26.6
  Route15 0.1: v212.76,26.6 212.76,20.8 211.76,19.8 211.76,17.47 J9.34
  Bottom 0.152: J3.34 211.46,8.89 211.46,15.24 J9.34
VSNSM_CH20  (via drill 0.2)
  Top 0.1: R98.1 217.81,27.64 217.76,27.6
  Top 0.15: 217.76,27.6 v217.76,26.6
  Route15 0.1: v217.76,26.6 217.76,20.8 216.76,19.8 216.76,17.55 J9.30
  Bottom 0.152: J3.30 216.53,8.89 216.53,15.24 J9.30
VSNSM_CH21  (via drill 0.2)
  Top 0.1: R100.1 233.26,27.9 233.37,27.8
  Top 0.15: 233.37,27.8 v233.97,27.8
  Route15 0.1: v233.97,27.8 233.97,17.43 J9.18
  Bottom 0.152: J3.18 231.78,8.89 231.78,15.24 J9.18
VSNSM_CH22  (via drill 0.2)
  Top 0.1: R102.1 235.66,27.9 235.76,27.8
  Top 0.15: 235.76,27.8 v236.6,27.8
  Route15 0.1: v236.6,27.8 236.6,17.49 J9.16
  Bottom 0.152: J3.16 234.31,8.89 234.31,15.24 J9.16
VSNSM_CH23  (via drill 0.2)
  Top 0.1: R104.1 238.26,27.9 238.37,27.8
  Top 0.15: 238.37,27.8 v239.16,27.8
  Route15 0.1: v239.16,27.8 239.16,17.55 J9.14
  Bottom 0.152: J9.14 236.85,15.24 236.85,8.89 J3.14
VSNSP0  (via drill 0.2)
  Top 0.1: U1.Z4 v123.3,52 | v22,24.8 21.09,24.8 R57.2
  Route2 0.1: v120.9,53.6 v22,53.6
  Route15 0.1: v123.3,52 122.6,52 121,53.6 v120.9,53.6 | v22,53.6 v22,24.8
  Bottom 0.1: C16.1 21.14,24.8 v22,24.8
VSNSP1  (via drill 0.2)
  Top 0.1: v29.64,24.8 28.7,24.8 R59.2
  Route2 0.1: v120.9,51.2 v29.64,51.2
  Route15 0.1: v29.64,51.2 v29.64,24.8
  Bottom 0.1: U1.X5 123.9,51.2 123.5,50.8 123.1,50.8 122.7,51.2 v120.9,51.2 | C18.1 28.73,24.8 v29.64,24.8
  other vias: 125.7,51.2
VSNSP2  (via drill 0.2)
  Top 0.1: C20.1 33.78,24.8 v34.63,24.8 34.03,24.8 33.91,24.93 R61.2
  Route2 0.1: v121.2,38.2 119.8,38.2 119.6,38 v34.34,38
  Route15 0.1: v34.34,38 34.34,26.3 34.63,26 v34.63,24.8 | v121.7,48.4 121.7,47.9 121.2,47.4 v121.2,38.2
  Bottom 0.1: v34.63,24.8 33.78,24.8 C20.1 | U1.Y7 123.7,48.4 v121.7,48.4
  other vias: 124.9,49.6
VSNSP3  (via drill 0.2)
  Top 0.1: R63.2 35.94,24.93 C22.1 | C22.1 R63.2 | C22.1 36.41,24.68 36.53,24.8 | v37.23,24.8 36.53,24.8 | 36.53,24.8 36.33,24.8 R63.2
  Route2 0.1: U1.X7 125.3,49.2 v120.9,49.2 | v120.6,37.7 119.9,37.7 119.6,37.4 v36.94,37.4
  Route15 0.1: v36.94,37.4 36.94,26.1 37.23,25.8 v37.23,24.8 | v120.9,49.2 120.9,48.8 120.6,48.5 v120.6,37.7
  Bottom 0.1: C22.1 36.32,24.8 v37.23,24.8
  other vias: 125.7,49.6
VSNSP4  (via drill 0.2)
  Top 0.1: v40.2,24.8 41.15,24.8 C24.1 R65.2
  Route2 0.1: v122.4,39.2 v40.2,39.2
  Route15 0.1: v40.2,39.2 v40.2,24.8 | U1.Y9 124.5,47.6 123.7,47.6 122.4,46.3 v122.4,39.2
  Bottom 0.1: v40.2,24.8 41.15,24.8 C24.1
  other vias: 124.9,48
VSNSP5  (via drill 0.2)
  Top 0.1: v57.5,24.8 56.84,24.8 56.83,24.81 56.64,24.81 R67.2
  Route2 0.1: U1.U9 126.9,47.6 126.3,47.6 126.1,47.4 126.1,43.9 125.6,43.4 v57.5,43.4
  Route15 0.1: v57.5,43.4 v57.5,24.8
  Bottom 0.1: v57.5,24.8 56.73,24.8 C26.1
  other vias: 127.3,48
VSNSP6  (via drill 0.2)
  Top 0.1: v59,26.2 59,24.95 R69.2
  Route2 0.1: v126.9,26.2 v59,26.2
  Route15 0.1: U1.R9 128.5,47.6 127.9,47.6 126.9,46.6 v126.9,26.2
  Bottom 0.1: C28.1 59.05,24.78 59,24.8 v59,26.2
  other vias: 128.9,48
VSNSP7  (via drill 0.2)
  Top 0.1: C30.1 61.72,24.8 v62.6,24.8 62.02,24.8 R71.2
  Route2 0.1: U1.R8 128.5,48.4 128.5,46.8 v127.3,45.6 | v127.3,31.2 v64.5,31.2 | v64.5,24.8 v62.6,24.8
  Route15 0.1: v127.3,45.6 v127.3,31.2 | v64.5,31.2 v64.5,24.8
  Bottom 0.1: C30.1 61.71,24.68 61.84,24.8 v62.6,24.8
  other vias: 128.9,48.8
VSNSP8  (via drill 0.2, 0.2 pad 0.25)
  Top 0.1: R73.2 C32.1 109.28,24.68 109.6,25
  Top 0.15: 109.6,25 v110.4,25
  Route2 0.1: v115,25 v110.4,25
  Route15 0.1: v115,48.8 v115,25
  Bottom 0.1: v110.4,25 109.54,25 C32.1 | U1.P4 128.8,52 128.4,52.4 127.7,52.4 127.3,52 126.1,52 125.7,52.4 122.7,52.4 122.2,51.9 118.1,51.9 v115,48.8
  other vias: 129.7,52
VSNSP9  (via drill 0.2)
  Top 0.1: C34.1 116.96,25 116.91,25 R75.2
  Top 0.15: v118,25 116.96,25
  Route2 0.1: U1.M5 130.9,50.8 130.1,50.8 129.3,50 129.3,46 v128.9,45.6 | v128.5,25 v118,25
  Route15 0.1: v128.9,45.6 128.9,25.4 v128.5,25
  Bottom 0.1: C34.1 117.2,25 v118,25
  other vias: 131.3,51.2
VSNSP10  (via drill 0.2)
  Top 0.1: v122,25.8 122,25.01 R77.2
  Route2 0.1: v128.5,25.8 v122,25.8
  Route15 0.1: U1.N7 130.1,50 129.5,50 129.3,49.8 129.3,46.4 128.9,46 128.7,46 128.5,45.8 v128.5,25.8
  Bottom 0.1: C36.1 122,24.68 v122,25.8
  other vias: 130.5,49.6
VSNSP11  (via drill 0.2)
  Top 0.1: 124.79,24.6 R79.2
  Top 0.15: v125.4,24.6 124.79,24.6
  Route2 0.1: U1.M7 130.9,49.2 v130.9,45.6 | v130.9,24.6 v125.4,24.6
  Route15 0.1: v130.9,45.6 v130.9,24.6
  Bottom 0.1: C38.1 124.8,24.6 v125.4,24.6
  other vias: 131.3,49.6
VSNSP12  (via drill 0.2)
  Top 0.1: v129.3,25.8 129.3,25.17 R81.2
  Route2 0.1: U1.N9 130.1,47.6 130.1,45.6 v129.3,44.8
  Route15 0.1: v129.3,44.8 v129.3,25.8
  Bottom 0.1: C40.1 129.3,25.16 v129.3,25.8
  other vias: 130.5,48
VSNSP13  (via drill 0.2)
  Top 0.1: v143.3,25 144.85,25 R83.2
  Route2 0.1: U1.K9 132.9,47.2 133.3,46.8 133.3,46.2 133.5,46 133.7,46 135.2,44.5 135.5,44.5 135.7,44.3 135.7,34.3 140.2,29.8 v143.3,29.8
  Route15 0.1: v143.3,29.8 143.3,28.3 143.2,28.2 143.2,27.7 143.3,27.6 v143.3,25
  Bottom 0.1: C42.1 R83.2 144.93,24.93 145,25 v143.3,25
  other vias: 132.9,48
VSNSP14  (via drill 0.2)
  Top 0.1: v145.7,25 147.39,25 R85.2 | U1.H9 134.9,47.6 134.9,46 135.6,45.3 137,45.3 137.7,44.6 v137.7,44
  Route2 0.1: v139.4,31.9 v145.7,31.9
  Route15 0.1: v137.7,44 137.7,43.6 138.5,42.8 138.5,32.8 v139.4,31.9 | v145.7,31.9 v145.7,25
  Bottom 0.1: C44.1 R85.2 147.6,25 v145.7,25
VSNSP15  (via drill 0.2)
  Top 0.1: R87.2 150.13,24.93 150.2,25 v148.4,25
  Route2 0.1: v139.9,26.8 140.6,26.8 141.2,26.2 147.2,26.2 v148.4,25
  Route15 0.1: U1.H8 135.7,47.6 135.7,45.9 136.6,45 137.8,45 138.4,44.4 138.4,43.4 138.9,42.9 138.9,33.2 139.9,32.2 v139.9,26.8
  Bottom 0.1: v148.4,25 150.18,25 C46.1
  other vias: 134.5,48.8
VSNSP16  (via drill 0.2, 0.2 pad 0.25)
  Top 0.1: 197.41,24.8 R89.2
  Top 0.15: v196.4,24.8 197.41,24.8
  Route2 0.1: U1.G4 136.5,53.2 139.5,53.2 141.1,54.8 v196.4,54.8
  Route15 0.1: v196.4,54.8 v196.4,24.8
  Bottom 0.1: C48.1 197.09,24.8 v196.4,24.8
  other vias: 135.3,52
VSNSP17  (via drill 0.2)
  Top 0.1: 205.03,24.8 R91.2
  Top 0.15: v204,24.8 205.03,24.8
  Route2 0.1: U1.E5 137.3,51.6 141.1,51.6 141.5,52 141.5,52.3 142,52.8 v204,52.8
  Route15 0.1: v204,52.8 v204,24.8
  Bottom 0.1: C50.1 204.99,24.8 v204,24.8
  other vias: 136.9,51.2
VSNSP18  (via drill 0.2)
  Top 0.1: 210.06,24.8 210.19,24.68 209.89,24.8 | 209.89,24.8 209.79,24.8 R93.2 210.06,24.8 | 209.89,24.8 210.06,24.8
  Top 0.15: v209,24.8 209.79,24.8
  Route2 0.1: U1.F7 136.5,49.2 137.9,49.2 138.1,49 138.1,48.6 138.3,48.4 141.5,48.4 141.9,48 v143.8,48 | v145.2,36.4 v209,36.4
  Route15 0.1: v143.8,48 145.4,46.4 145.4,42 145.2,41.8 v145.2,36.4 | v209,36.4 v209,24.8
  Bottom 0.1: R93.2 C52.1 209.99,24.8 v209,24.8
  other vias: 136.1,49.6
VSNSP19  (via drill 0.2)
  Top 0.1: 212.72,24.68 212.6,24.8 212.6,24.81 R95.2
  Top 0.15: v211.8,24.8 212.6,24.8
  Route2 0.1: v143.6,37 v211.8,37
  Route15 0.1: U1.E7 137.3,49.2 141.2,49.2 141.6,48.8 141.6,47.2 143.6,45.2 v143.6,37 | v211.8,37 v211.8,24.8
  Bottom 0.1: C54.1 212.39,24.8 v211.8,24.8
  other vias: 136.9,49.6
VSNSP20  (via drill 0.2)
  Top 0.1: U1.F9 136.5,47.6 136.5,46.2 136.9,45.8 139.9,45.8 140.9,44.8 v140.9,44 | 217.81,24.68 217.68,24.8 v216.76,24.8 | 217.68,24.8 R97.2
  Top 0.15: v216.76,24.8 217.68,24.8
  Route2 0.1: v140.9,38.8 v216.76,38.8
  Route15 0.1: v140.9,44 v140.9,38.8 | v216.76,38.8 v216.76,24.8
  Bottom 0.1: 217.5,24.8 217.59,24.8 | 217.59,24.8 217.68,24.8 R97.2 217.5,24.8 | C56.1 217.59,24.8 | 217.5,24.8 v216.76,24.8
VSNSP21  (via drill 0.2)
  Top 0.1: R99.2 232.9,24.93 232.76,24.8 v231.97,24.8
  Route2 0.1: v142.4,40.6 v231.3,40.6
  Route15 0.1: U1.C9 139.6,46.9 139.6,46.2 139.8,46 141,46 142.4,44.6 v142.4,40.6 | v231.3,40.6 231.3,25.4 v231.97,24.8
  Bottom 0.1: v231.97,24.8 232.92,24.8 C58.1
  other vias: 138.5,48
VSNSP22  (via drill 0.2)
  Top 0.1: R101.2 235.4,24.8 v234.66,24.8
  Route2 0.1: U1.A9 140.5,48 140.9,47.6 v146.2,47.6 | v146.6,41.8 v235.06,41.8
  Route15 0.1: v146.2,47.6 146.6,47.2 v146.6,41.8 | v235.06,41.8 235.06,25.2 v234.66,24.8
  Bottom 0.1: v234.66,24.8 235.46,24.8 C60.1
  other vias: 140.1,48
VSNSP23  (via drill 0.2)
  Top 0.1: R103.2 238,24.8 v237.16,24.8 | U1.A8 v140.9,48.8
  Route2 0.1: v140.9,48.8 141.6,48.8 142,48.4 v237.8,48.4
  Route15 0.1: v237.8,48.4 237.8,25.4 v237.16,24.8
  Bottom 0.1: v237.16,24.8 238,24.8 C62.1
VSNSP_CH0
  Top 0.1: J7.45 R57.1
  Top 0.152: J1.45 22.23,11.43 22.23,17.78 J7.45
VSNSP_CH1
  Top 0.1: J7.39 R59.1
  Top 0.152: J1.39 29.84,11.43 29.84,17.78 J7.39
VSNSP_CH2
  Top 0.1: J7.35 R61.1
  Top 0.152: J1.35 34.92,11.43 34.92,17.78 J7.35
VSNSP_CH3
  Top 0.1: J7.33 R63.1
  Top 0.152: J1.33 37.47,11.43 37.47,17.78 J7.33
VSNSP_CH4
  Top 0.1: J7.29 R65.1
  Top 0.152: J1.29 42.55,11.43 42.55,17.78 J7.29
VSNSP_CH5
  Top 0.1: J7.17 R67.1
  Top 0.152: J1.17 57.78,11.43 57.78,17.78 J7.17
VSNSP_CH6
  Top 0.1: J7.15 R69.1
  Top 0.152: J1.15 60.33,11.43 60.33,17.78 J7.15
VSNSP_CH7
  Top 0.1: R71.1 J7.13
  Top 0.152: J1.13 62.87,11.43 62.87,17.78 J7.13
VSNSP_CH8
  Top 0.15: R73.1 J8.45
  Top 0.152: J2.45 110.49,11.43 110.49,17.78 J8.45
VSNSP_CH9
  Top 0.15: J8.39 R75.1
  Top 0.152: J2.39 118.11,11.43 118.11,17.78 J8.39
VSNSP_CH10
  Top 0.15: R77.1 J8.35
  Top 0.152: J2.35 123.19,11.43 123.19,17.78 J8.35
VSNSP_CH11
  Top 0.15: R79.1 J8.33
  Top 0.152: J2.33 125.73,11.43 125.73,17.78 J8.33
VSNSP_CH12
  Top 0.1: R81.1 129.5,23.3 129.2,23 | 129.5,19.09 J8.29
  Top 0.15: 129.2,23 129.2,20.4 129.5,20.1 129.5,19.09
  Top 0.152: J2.29 130.81,11.43 130.81,17.78 J8.29
VSNSP_CH13
  Top 0.15: R83.1 J8.17
  Top 0.152: J2.17 146.05,11.43 146.05,17.78 J8.17
VSNSP_CH14
  Top 0.15: R85.1 J8.15
  Top 0.152: J2.15 148.59,11.43 148.59,17.78 J8.15
VSNSP_CH15
  Top 0.15: R87.1 J8.13
  Top 0.152: J2.13 151.13,11.43 151.13,17.78 J8.13
VSNSP_CH16
  Top 0.15: J9.45 R89.1
  Top 0.152: J3.45 198.75,11.43 198.75,17.78 J9.45
VSNSP_CH17
  Top 0.15: J9.39 R91.1
  Top 0.152: J3.39 206.38,11.43 206.38,17.78 J9.39
VSNSP_CH18
  Top 0.15: J9.35 R93.1
  Top 0.152: J3.35 211.46,11.43 211.46,17.78 J9.35
VSNSP_CH19
  Top 0.15: J9.33 R95.1
  Top 0.152: J3.33 214,11.43 214,17.78 J9.33
VSNSP_CH20
  Top 0.15: J9.29 R97.1
  Top 0.152: J3.29 219.07,11.43 219.07,17.78 J9.29
VSNSP_CH21
  Top 0.15: J9.17 R99.1
  Top 0.152: J3.17 234.31,11.43 234.31,17.78 J9.17
VSNSP_CH22
  Top 0.15: R101.1 J9.15
  Top 0.152: J3.15 236.85,11.43 236.85,17.78 J9.15
VSNSP_CH23
  Top 0.15: R103.1 J9.13
  Top 0.152: J3.13 239.4,11.43 239.4,17.78 J9.13
WP  (via drill 0.2, 0.2 pad 0.25)
  Top 0.1: U1.A2 v140.9,53.6
  Route2 0.1: v140.9,56.8 v134.5,56.8 v128.9,56.8 v99,56.8
  Route15 0.1: v140.9,53.6 v140.9,56.8 | v99,56.8 99,74.14 JP7.1
  Bottom 0.1: R56.1 102.08,73.9 100.3,73.9 100,74.2 JP7.1 | v134.5,56.8 134.5,56 134.9,55.6 134.9,54 U1.H2 | U1.R2 128.5,54 128.5,54.8 128.9,55.2 v128.9,56.8
  other vias: 128.9,53.6 134.5,53.6

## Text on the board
tPlace: Write-Protect | GND | SDA | SCL | ON | SHARE_CLK | GND | RUN | RUN | OFF | PWRGD | ALERTB | FAULTBZ0 | FAULTBZ1 | RESET | ASEL1 | ASEL0 | ASEL1 | ASEL0 | ASEL1 | ASEL0 | OFF | OFF | HIGH | CTRL0 | CTRL1 | FLOAT | LOW | U1 | DevA | DevB | DevC | FAULTB00 | FAULTB01 | FAULTB10 | FAULTB11 | Demo Circuit 3094A | LTC2980-24 | Pairs with 3x DC1361B Boards | 24-CH Digital Power System Manager | VIN | CH0 - CH7 | CH8 - CH15 | CH16 - CH23 | Sense Only | GND | GND | 49 | 47 | 43 | 39 | 35 | 31 | 27 | 23 | 19 | 15 | 11 | 7 | 3 | 49 | 47 | 43 | 39 | 35 | 31 | 27 | 23 | 19 | 15 | 11 | 7 | 3 | 49 | 47 | 43 | 39 | 35 | 31 | 27 | 23 | 19 | 15 | 11 | 7 | 3 | 54 | 50 | 46 | 42 | 38 | 34 | 30 | 26 | 22 | 18 | 14 | 10 | 6 | 2 | GND | 54 | 50 | 46 | 42 | 38 | 34 | 30 | 26 | 22 | 18 | 14 | 10 | 6 | 2 | GND | 54 | 50 | 46 | 42 | 38 | 34 | 30 | 26 | 22 | 18 | 14 | 10 | 6 | 2
bPlace: Rev 1 | mtp
d_FabDrawing: 3.40" | 0.00" | 0.00" | 10.40" | DRILL TABLE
